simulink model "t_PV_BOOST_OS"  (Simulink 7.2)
settings: Solver=ode3  StartTime=0.0  StopTime=1  FixedStep=10e-6  MaxStep=1e-5  RelTol=1e-5  AbsTol=1e-5

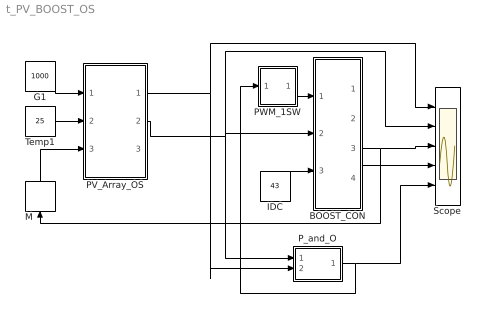
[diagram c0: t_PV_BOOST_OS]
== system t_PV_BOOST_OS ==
  BOOST_CON : Subsystem  mask{L1=10e-3, IL0=50, C1=5e-3, UC0=1000, R1=1e5}
      mask prompts: L1 "Inductance L1"; IL0 "Initial Current"; C1 "Capacitance"; UC0 "Initial Voltage"; R1 "Load Resistance"
      mask help: Open Source boost Converter Input Vector u: u[0]= T1.gate u[1]= E.v u[2]= IDC.i Output Vector y: y[0]= T1.I y[1]= D1.I y[2]= L1.I y[3]= C1.V Parameter Vector p: p[0]= L1.L p[1]= L1.iL0 p[2]= C1.C p[3]= C1.vC0 p[4]= R1.r You can pause the simulation during running, change the Parameters you want and continue the Simulation
  G1 : Constant  Value=1000  OutDataType=sfix(16)  OutScaling=2^0
  IDC : Constant  Value=43  OutDataType=sfix(16)  OutScaling=2^0
  M : Memory  Orientation=up
  PV_Array_OS : Subsystem  mask{Isc0=5.28, Ud0=44.5, Ki=2e-3, Kv=-0.1558, n=1.0, RS=0.7, RP=400, NC=72, NMs=20, NMp=15, C=1e-4, vC0=0, RL=10000}
      mask prompts: Isc0 "Short Circuit Current at STC Isc0/Module"; Ud0 "Open Circuit Voltage at STC Ud0/Module"; Ki "Short Circuit Current Temp Coeff. Ki/Module"; Kv "Open Circuit Voltage Temp. Coeff. Kv/Module"; n "Diode Idealty Factor n"; RS "Series Resistance Rs"; RP "Parallel Resistance RP"; NC "Number Cells"; NMs "Number Series Modules"; NMp "Number Parallel Modules"; C "Load Capacitor"; vC0 "init Cap Voltage"; RL "Load Res."
      mask help: PV_Array_OS with parameters: N_Cells/Module (NC), N_Series connected Module (NMs) and N_parallel connected Module (NMp) Input Vector u: u[0]=G u[1]=T u[2]=ILd Output Vector y: y[0]=PV.I y[1]=PV.V y[2]=C.I Parameter Vector p: p[0]=Isc0 p[1]=Ud0 p[2]=Ki p[3]=Kv p[4]=n p[5]=RS p[6]=RP p[7]=NC p[8]=NMs p[9]=NMp p[10]=C p[11]=vC0 p[12]=RL You can pause the simulation during running, change the Parameters you want and continue the Simulation
  PWM_1SW : Subsystem  mask(PWMtr){FS=1e3}
      mask prompts: FS "Frequency"
  P_and_O : Subsystem  mask{DeltaD=0.00001}
      mask help: MPPT controller based on the Perturb & Observe algorithm. D output = Duty cycle of the boost converter (value between 0 and 1) DeltaD = 0.0001; Increment value used to increase/decrease the duty cycle D
  Scope : Scope  NumInputPorts=5
  Temp1 : Constant  Value=25  OutDataType=sfix(16)  OutScaling=2^0
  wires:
  G1/1 -> PV_Array_OS/1(G)
  Temp1/1 -> PV_Array_OS/2(Temp)
  PWM_1SW/1(Out1) -> BOOST_CON/1(sw)
  P_and_O/1(D) -> PWM_1SW/1(In1), Scope/5
  PV_Array_OS/2(PV_V) -> BOOST_CON/2(E), P_and_O/1(V), Scope/2
  BOOST_CON/3(iL) -> M/1, Scope/3
  PV_Array_OS/1(PV_I) -> P_and_O/2(I), Scope/1
  BOOST_CON/4(vC) -> Scope/4
  M/1 -> PV_Array_OS/3(ILd)
  IDC/1 -> BOOST_CON/3(IDC)

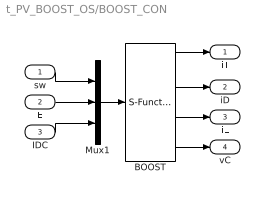
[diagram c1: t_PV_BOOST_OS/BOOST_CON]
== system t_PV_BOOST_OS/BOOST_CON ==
  sw : Inport  OutDataType=sfix(16)  OutScaling=2^0
  E : Inport  Port=2  OutDataType=sfix(16)  OutScaling=2^0
  IDC : Inport  Port=3  OutDataType=sfix(16)  OutScaling=2^0
  BOOST : S-Function  FunctionName=s_boost_OS  Parameters="[L1  IL0  C1   UC0  R1]"  EnableBusSupport=off
  Mux1 : Mux  Inputs=3
  iT : Outport  OutDataType=sfix(16)  OutScaling=2^0
  iD : Outport  Port=2  OutDataType=sfix(16)  OutScaling=2^0
  iL : Outport  Port=3  OutDataType=sfix(16)  OutScaling=2^0
  vC : Outport  Port=4  OutDataType=sfix(16)  OutScaling=2^0
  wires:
  IDC/1 -> Mux1/3
  BOOST/4 -> vC/1
  BOOST/3 -> iL/1
  BOOST/2 -> iD/1
  BOOST/1 -> iT/1
  E/1 -> Mux1/2
  sw/1 -> Mux1/1
  Mux1/1 -> BOOST/1

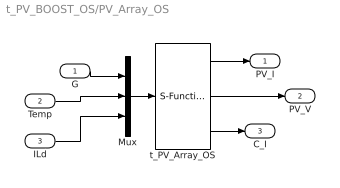
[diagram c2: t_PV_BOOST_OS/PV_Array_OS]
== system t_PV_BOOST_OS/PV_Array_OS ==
  G : Inport
  Temp : Inport  Port=2
  ILd : Inport  Port=3
  Mux : Mux  Inputs=3
  t_PV_Array_OS : S-Function  FunctionName=s_PV_Array_OS  Parameters="[Isc0  Ud0  Ki  Kv  n    RS  RP NC  NMs NMp C  vC0  RL]"  EnableBusSupport=off
  PV_I : Outport
  PV_V : Outport  Port=2
  C_I : Outport  Port=3
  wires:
  Mux/1 -> t_PV_Array_OS/1
  G/1 -> Mux/1
  Temp/1 -> Mux/2
  ILd/1 -> Mux/3
  t_PV_Array_OS/1 -> PV_I/1
  t_PV_Array_OS/2 -> PV_V/1
  t_PV_Array_OS/3 -> C_I/1

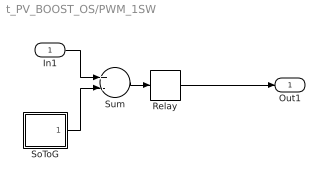
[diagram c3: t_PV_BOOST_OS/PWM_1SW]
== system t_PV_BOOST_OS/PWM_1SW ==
  In1 : Inport  OutDataType=sfix(16)  OutScaling=2^0
  Relay : Relay  OutDataType=sfix(16)  OutScaling=2^0
  SoToG : Subsystem  mask(SoToG){T=1/FS}
      mask prompts: T "Period Time"
  Sum : Sum  Inputs=+-  OutDataType=sfix(16)  OutScaling=2^0
  Out1 : Outport  InitialOutput=0
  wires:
  Relay/1 -> Out1/1
  SoToG/1(O) -> Sum/2
  In1/1 -> Sum/1
  Sum/1 -> Relay/1

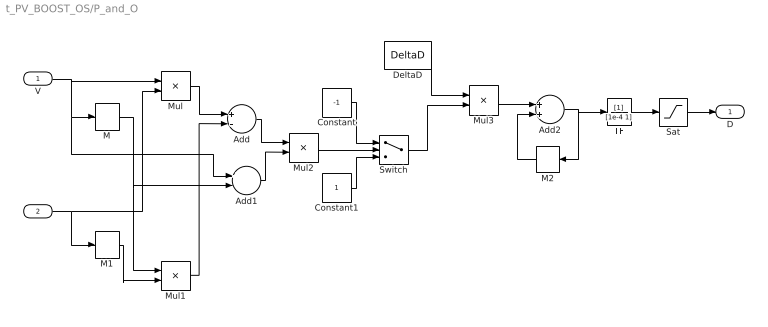
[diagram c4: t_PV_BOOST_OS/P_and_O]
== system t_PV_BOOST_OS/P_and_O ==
  V : Inport  OutDataType=sfix(16)  OutScaling=2^0
  I : Inport  Port=2  OutDataType=sfix(16)  OutScaling=2^0
  Add : Sum  Inputs=+-  OutDataType=sfix(16)  OutScaling=2^-10
  Add1 : Sum  Inputs=+-  OutDataType=sfix(16)  OutScaling=2^-10
  Add2 : Sum  OutDataType=sfix(16)  OutScaling=2^-10
  Constant : Constant  Value=-1  OutDataType=sfix(16)  OutScaling=2^0
  Constant1 : Constant  OutDataType=sfix(16)  OutScaling=2^0
  DeltaD : Constant  Value=DeltaD  OutDataType=sfix(16)  OutScaling=2^0
  M : Memory
  M1 : Memory
  M2 : Memory  Orientation=left
  Mul{,1..3} (4 alike) : Product  Inputs=**  OutDataType=sfix(16)  OutScaling=2^-10
  Sat : Saturate  UpperLimit=1  LowerLimit=0  OutDataType=sfix(16)  OutScaling=2^0
  Switch : Switch  OutDataType=sfix(16)  OutScaling=2^0
  TF : TransferFcn  Denominator=[1e-4 1]
  D : Outport  OutDataType=sfix(16)  OutScaling=2^0
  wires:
  Sat/1 -> D/1
  TF/1 -> Sat/1
  M2/1 -> Add2/2
  Add2/1 -> TF/1, M2/1
  Mul3/1 -> Add2/1
  DeltaD/1 -> Mul3/1
  Switch/1 -> Mul3/2
  Constant1/1 -> Switch/3
  Constant/1 -> Switch/1
  Mul2/1 -> Switch/2
  Add1/1 -> Mul2/2
  Add/1 -> Mul2/1
  Mul1/1 -> Add/2
  Mul/1 -> Add/1
  M1/1 -> Mul1/2
  M/1 -> Add1/2, Mul1/1
  V/1 -> Add1/1, M/1, Mul/1
  I/1 -> M1/1, Mul/2

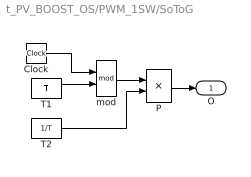
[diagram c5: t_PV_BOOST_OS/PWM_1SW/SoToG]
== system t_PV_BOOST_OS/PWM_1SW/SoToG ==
  Clock : Clock
  P : Product  OutDataType=sfix(16)  OutScaling=2^0
  T1 : Constant  Value=T  OutDataType=sfix(16)  OutScaling=2^0
  T2 : Constant  Value=1/T  OutDataType=sfix(16)  OutScaling=2^0
  mod : Math  Operator=mod
  O : Outport
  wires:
  P/1 -> O/1
  mod/1 -> P/1
  T2/1 -> P/2
  T1/1 -> mod/2
  Clock/1 -> mod/1
